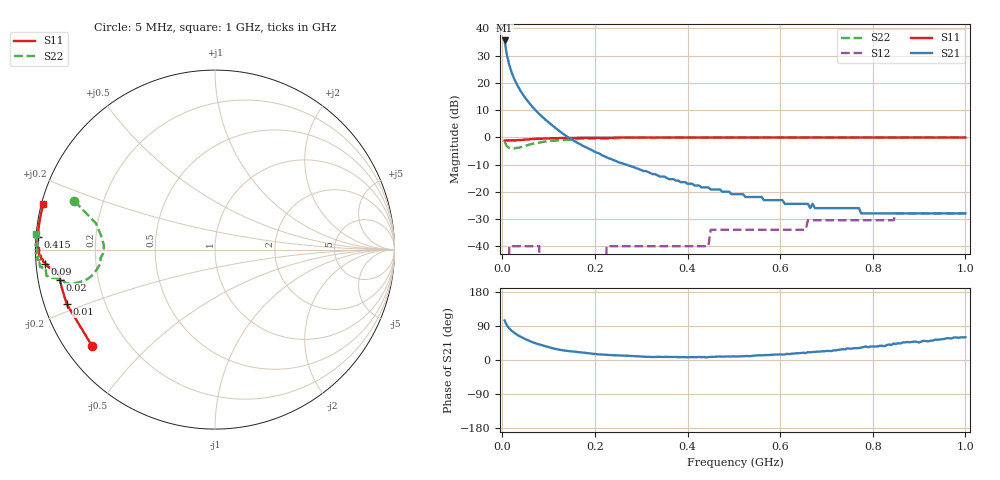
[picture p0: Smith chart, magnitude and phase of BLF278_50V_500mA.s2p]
! Filename:  BLF278_50V_500mA.s2p
! Philips part #: BLF278  !date: 22-05-2003
!Vdd=50V ; Idq=500mA
!D:\Vee measurements\measurement data\VDMOST\BLF278\50V_500mA_#1
# HZ S MA R 50
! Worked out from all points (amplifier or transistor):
!   200 points, 5 MHz to 1 GHz, reference 50 ohm
!   highest |S21| = 35.6 dB at 5 MHz (marker M1)
!   |S21| within 3 dB of that: start of sweep to 7.756 MHz
!   S11 on the Smith chart (normalised r, x): 5 MHz: 0.08, -0.34; 10 MHz: 0.07, -0.18; 20 MHz: 0.06, -0.10; 90 MHz: 0.03, -0.04; 415 MHz: 0.01, +0.04; 1 GHz: 0.01, +0.13
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5000000  0.87 -142.1  60.05 104.3  0 -19.4  0.83 160.9
1e7  0.88 -159.8  32.09 91.4  0 11.2  0.68 167.5
1.5e7  0.88 -166.1  21.47 83.3  0.01 16.3  0.64 172.9
2e7  0.88 -169.0  15.7 77.3  0.01 13.4  0.62 177.6
2.5e7  0.88 -170.4  12.25 72.8  0.01 8.8  0.62 -178.5
3e7  0.88 -171.2  9.98 68.4  0.01 3.4  0.64 -175.8
3.5e7  0.89 -171.8  8.27 64.4  0.01 -0.9  0.64 -173.5
4.5e7  0.9 -172.6  6.01 57.9  0.01 -7.4  0.68 -169.4
6e7  0.92 -173.5  4.08 49.6  0.01 -15.0  0.74 -166.8
8e7  0.94 -174.7  2.66 41.0  0.01 -19.8  0.8 -166.5
8.5e7  0.94 -175.0  2.43 39.3  0 -19.9  0.81 -166.6
9e7  0.95 -175.2  2.22 37.5  0 -19.7  0.83 -166.7
1.25e8  0.97 -176.9  1.27 26.8  0 -1.9  0.88 -169.4
1.75e8  0.98 -178.7  0.69 19.5  0 65.3  0.94 -170.8
2.2e8  0.98 180.0  0.45 13.8  0 82.7  0.95 -173.3
2.25e8  0.98 179.8  0.43 13.4  0.01 83.6  0.95 -173.5
3.4e8  0.99 177.3  0.19 8.4  0.01 89.4  0.98 -176.3
4.15e8  0.99 175.8  0.13 7.5  0.01 91.3  0.98 -177.8
5.05e8  0.99 174.1  0.09 9.2  0.02 91.4  0.99 -179.3
6.7e8  0.99 171.2  0.06 21.0  0.03 92.4  1 178.5
8.35e8  0.99 168.3  0.04 41.0  0.03 94.6  0.99 177.0
1e9  0.99 165.2  0.04 60.3  0.04 94.1  1 175.0
